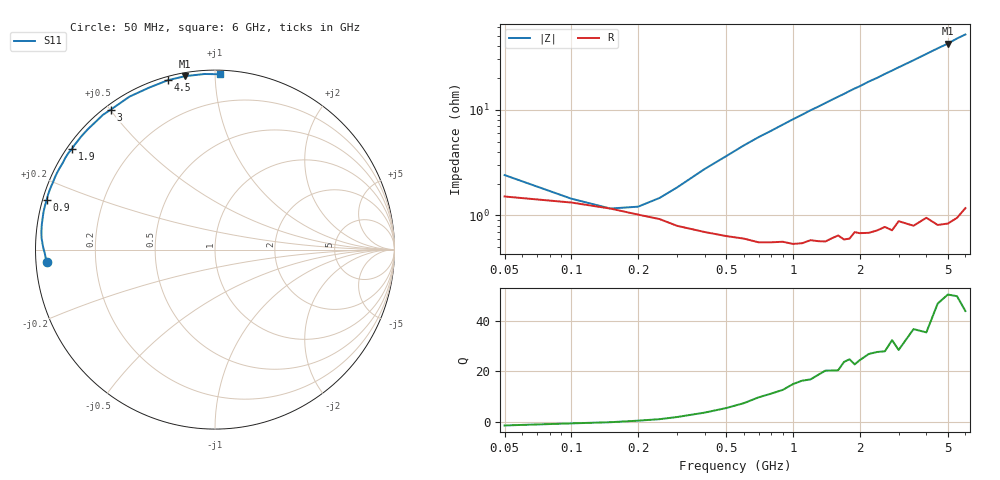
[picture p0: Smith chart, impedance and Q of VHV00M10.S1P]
! Infineon Technologies  Discrete & RF Semiconductors
! BB 814
! Si Tuning Diode in SOT23
! VR =
! S-Parameters:  July  1999
# GHz  S  MA  R  50
!  f  S11
! GHz  MAG  ANG
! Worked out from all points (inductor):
!   34 points, 50 MHz to 6 GHz, reference 50 ohm
!   read as one part to ground: L = 1.17 nH near 400 MHz
!   highest Q = 49.6 at 5 GHz (marker M1), where L = 1.34 nH
!   S11 on the Smith chart (normalised r, x): 50 MHz: 0.03, -0.04; 900 MHz: 0.01, +0.14; 1.9 GHz: 0.01, +0.32; 3 GHz: 0.02, +0.50; 4.5 GHz: 0.02, +0.76; 6 GHz: 0.02, +1.03
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0.05  0.9414 -175.7
0.1  0.9484 -178.7
0.2  0.9601 178.5
0.3  0.9686 176.2
0.4  0.9726 173.9
0.5  0.9749 171.8
0.7  0.9782 167.5
0.8  0.9783 165.6
0.9  0.9781 163.6
1.1  0.979 159.7
1.3  0.9784 155.9
1.5  0.9773 152.1
1.6  0.9761 150.3
1.7  0.9783 148.5
1.8  0.9781 146.6
1.9  0.975 144.8
2  0.9758 143.2
2.2  0.9762 139.5
2.4  0.9754 136.4
2.6  0.9741 132.9
2.8  0.9765 129.8
3  0.9722 126.6
3.5  0.9765 119.2
4  0.9742 112.1
4.5  0.9796 105.5
5  0.9806 99.7
5.5  0.9801 93.4
6  0.9774 88.4
